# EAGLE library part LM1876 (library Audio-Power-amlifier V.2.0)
The LM1876 is a stereo audio amplifier capable of delivering typically 20W per channel of continuous average output power into a 4Ω or 8Ω load with less than 0.1% THD+N. Each amplifier has an independent smooth transition fade-in/out mute and a power conserving standby mode which can be controlled by external logic.
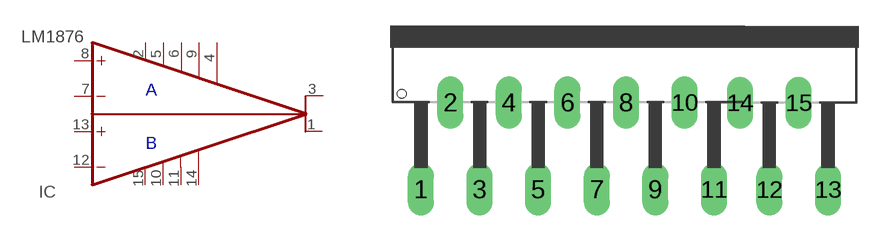
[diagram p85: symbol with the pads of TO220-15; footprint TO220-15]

Designator prefix IC

## LM1876  [TO220-15]
1  OUTB  out
2  VCCA  pwr
3  OUTA  out
4  VEE  pwr
5  GNDA  pwr
6  MUTE_A
7  -INA  in
8  +INA  in
9  STANDBY_A
10  GNDB  pwr
11  MUTE_B
12  -INB  in
13  +INB  in
14  STANDBY_B
15  VCCB  pwr

## Footprint TO220-15 (pad centres in mm)
drill 1.016 long: 1 0.381,1.905; 2 2.083,6.96; 3 3.785,1.905; 4 5.486,6.96; 5 7.188,1.905; 6 8.89,6.96; 7 10.592,1.905; 8 12.294,6.96; 9 13.995,1.905; 10 15.697,6.96; 11 17.399,1.905; 12 20.615,1.895; 13 24.019,1.895; 14 18.914,6.95; 15 22.317,6.95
